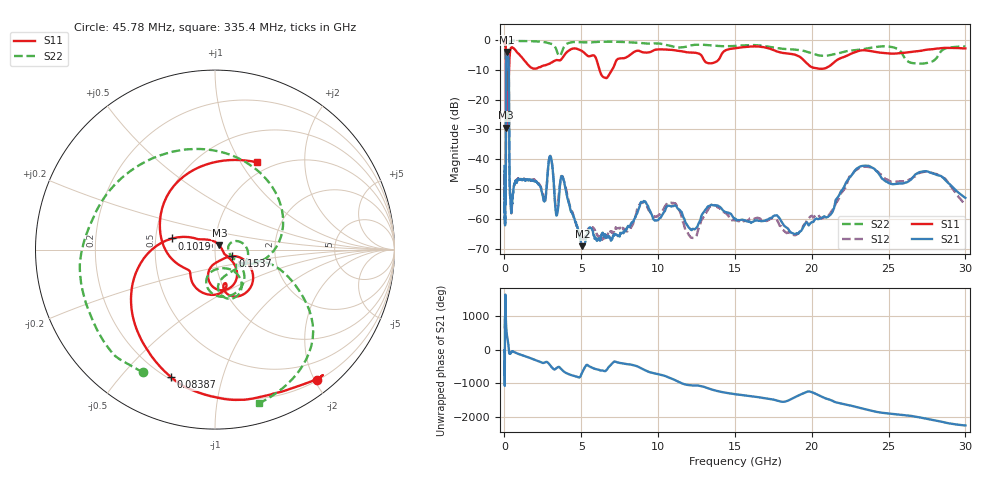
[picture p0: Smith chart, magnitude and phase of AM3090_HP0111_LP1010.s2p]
! Date/Time: Thu, Feb 28, 2019 2:01 PM
! Network Analyzer: Agilent Technologies E8364B Rev: A.07.50.67
! Sweep from 0.010 to 30.000 GHz, 1601 Points, Sweep Type: LOG
! Power Supply: 5.023 V, 0.002 A
# Hz S DB R 50
!freq MagS11 AngS11 MagS21 AngS21 MagS12 AngS12 MagS22 AngS22
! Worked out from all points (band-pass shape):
!   1601 points, 10 MHz to 30 GHz, reference 50 ohm
!   highest |S21| = -4.05 dB at 165.6 MHz (marker M1); lowest = -69.2 dB at 5.077 GHz (marker M2)
!   |S21| within 3 dB of the highest: 114.4 MHz to 271.9 MHz (157.5 MHz wide, 81.5 % of centre)
!   lowest |S11| = -29.4 dB at 109.9 MHz (marker M3), VSWR 1.07, Z = 52.5 + j2.42 ohm
!   |S11| at or under -10 dB: 100.6 MHz to 297.5 MHz (196.9 MHz wide, 98.9 % of centre); 6.184 GHz to 7.009 GHz (824.4 MHz wide, 12.5 % of centre)
!   |S22| runs from -22.7 to -0.2 dB; largest |S21 - S12| = 0.012
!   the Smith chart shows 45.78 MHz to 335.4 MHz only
!   S11 on the Smith chart (normalised r, x): 45.78 MHz: 0.21, -2.03; 83.87 MHz: 0.21, -0.69; 101.9 MHz: 0.61, +0.08; 153.7 MHz: 1.21, -0.09; 335.4 MHz: 0.86, +1.18
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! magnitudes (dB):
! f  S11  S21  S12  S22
! 10 MHz  -0.2  -42.3  -45.0  -0.7
! 38.04 MHz  -0.5  -60.5  -58.9  -1.5
! 45.78 MHz  -0.7  -51.3  -54.2  -2.0
! 83.87 MHz  -2.5  -50.9  -52.6  -4.7
! 101.9 MHz  -12.2  -17.3  -17.3  -11.4
! 109.9 MHz  -29.4  -8.8  -8.8  -22.2
! 125.2 MHz  -12.8  -5.5  -5.5  -15.4
! 144.7 MHz  -23.1  -4.4  -4.4  -16.4
! 153.7 MHz  -19.7  -4.1  -4.1  -16.3
! 165.6 MHz  -12.5  -4.1  -4.0  -13.4
! 276 MHz  -14.2  -7.7  -7.7  -16.0
! 335.4 MHz  -5.4  -47.5  -48.6  -1.0
! 550.5 MHz  -2.7  -51.7  -51.4  -0.3
! 2.084 GHz  -9.6  -47.5  -47.8  -0.5
! 2.623 GHz  -8.5  -53.9  -54.4  -0.7
! 3.002 GHz  -7.7  -39.0  -39.1  -1.2
! 3.385 GHz  -6.7  -58.9  -57.6  -3.4
! 5.077 GHz  -3.8  -69.2  -66.4  -0.8
! 7.926 GHz  -5.8  -63.3  -64.2  -0.7
! 18.84 GHz  -4.8  -65.0  -65.4  -3.2
! 23.48 GHz  -3.5  -42.2  -42.5  -3.0
! 30 GHz  -2.8  -52.9  -55.4  -2.2
